(* Logix 5000 Rung export; software revision 16.04 *)

MODULES
   PBS : vendor None type None code None
   Local : vendor None type None code None
END_MODULES

TYPE ILX69PBS_UTIL_AOI :
STRUCT
   InputArray : ILX69PBS_UTIL_AOI_INPUT_ARRAY;   // Input from Module
   OutputArray : ILX69PBS_UTIL_AOI_OUTPUT_ARRAY;   // Output to Module
   InputSize : INT;
   OutputSize : INT;
   InputDataSize : INT;
   InputCopyLength : INT;
   OutputDataSize : INT;
   OutputCopyLength : INT;
   OutputCopyLastLength : INT;
   OutputConnectionSize : INT;
   UTILOutputCopyLength : INT;
   PreviousBPActivityCounter : INT;
   ReadReqMasterLengthDINT : DINT;
   AlarmReqMasterLengthDINT : DINT;
END_STRUCT
END_TYPE

TYPE ILX69PBS_UTIL_MSG_SETEXTDIAG_REQUEST :   // Slave Diagnostic Request
STRUCT
   Status : DINT;   // Slave Status
   Command : DINT;   // Message Command. Set to 0x040E
   ExtendedDiagnosticOverflow : SINT;   // Set bit 0 to indicate that more diagnostic data is available as diagnostic data can be transferred with Data below
   Reserved1 : SINT;   // Reserved
   Reserved2 : SINT;
   Reserved3 : SINT;
   ExtendedDiagData : SINT[237];   // Diagnostic Data to be transferred
END_STRUCT
END_TYPE

TYPE ILX69PBS_DPV1_READ_RESPONE_TO_MASTER :   // DPV1 Read Response to Master
STRUCT
   Initiate : BOOL;   // Initiate a response to the Masters DPV1 read request with the associated read data.
   InhibitAutoInitiate : BOOL;   // Inhibitit Automatically Initiating a response. Master Address, Slot, Index, Length and data are copied to response.
   Slot : SINT;   // Place Requested Slot Number
   Index : SINT;   // Place Requested Index
   Length : SINT;   // Place Requested Data Length
   Data : SINT[240];   // Place Requested Data
END_STRUCT
END_TYPE

TYPE ILX69PBS_DPV1_WRITE :   // DPV1 Write
STRUCT
   RequestFromMaster : ILX69PBS_DPV1_WRITE_REQ_FROM_MASTER;   // DPV1 Write Request from Master
   ResponseToMaster : ILX69PBS_DPV1_WRITE_RESPONSE_TO_MASTER;   // DPV1 Write Response to Master
   MSGStatus : ILX69PBS_MESSAGE_STATUS;   // DPV1 Write MSG Status
END_STRUCT
END_TYPE

TYPE ILX69PBS_UTIL_AOI_DEV_STATUS_REGISTER :   // Device Status Register
STRUCT
   Reserved0 : BOOL;   // Reserved
   Reserved1 : BOOL;   // Reserved
   Reserved2 : BOOL;   // Reserved
   Reserved3 : BOOL;   // Reserved
   Reserved4 : BOOL;   // Reserved
   Communication : BOOL;   // Communication
   Running : BOOL;   // Running
   Ready : BOOL;   // Ready
   Reserved5 : SINT;   // Reserved
   Reserved6 : SINT;   // Reserved
   Reserved7 : SINT;   // Reserved
END_STRUCT
END_TYPE

TYPE ILX69PBS_UTIL_MSG_DPV1_ALARM :   // DPV1 Alarm MSG Status, Source and Destination
STRUCT
   Source : ILX69PBS_UTIL_MSG_DPV1_ALARM_REQUEST;   // Source. Request from Master
   Destination : ILX69PBS_UTIL_MSG_DPV1_ALARM_RESPONSE;   // Destination. Response to Master
END_STRUCT
END_TYPE

TYPE ILX69PBS_UTIL_MSG_DPV1_WRITE_RESPONSE :   // DPV1 Write Response
STRUCT
   Status : DINT;   // Status
   Command : DINT;   // Message Command. Set to 0x0487
   SlotNumber : SINT;   // Slot Number
   Index : SINT;   // Index
   Length : SINT;   // Length
   Reserved1 : SINT;   // Reserved
   ErrorDecode : SINT;   // Error Code Classifying Fault
   ErrorCode1 : SINT;   // Detailed Error Code
   ErrorCode2 : SINT;   // User Specific Error Code
   Reserved2 : SINT;   // Reserved
   Data : SINT[240];   // Write Data
END_STRUCT
END_TYPE

TYPE ILX69PBS_UTIL_MSG_SETEXTDIAG_RESPONSE :   // Slave Diagnostic Response
STRUCT
   Status : DINT;   // Slave Status
   Command : DINT;   // Message Command. Reposnds with 0x040F
END_STRUCT
END_TYPE

TYPE ILX69PBS_CONTROL :
STRUCT
   ColdBoot : BOOL;   // Cold Boot Reset
   GetExtendedStatus : ILX69PBS_CONTROL_GETEXTENDEDDIAG;   // Get Extended Status Information Select
   SetExtendedDiagnostic : ILX69PBS_CONTROL_SETEXTENDEDDIAG;   // Set Slave Diagnostic Extended Data
END_STRUCT
END_TYPE

TYPE ILX69PBS_UTIL_MSG_DPV1_READ_REQUEST :   // DPV1 Read Request MSG Structure
STRUCT
   Status : DINT;   // Status
   Command : DINT;   // Message Command. Set to 0x0485
   SlotNumber : SINT;   // Slot Number
   Index : SINT;   // Index
   Length : SINT;   // Length
   Reserved1 : SINT;   // Reserved
   ErrorDecode : SINT;   // Error Code Classifying Fault
   ErrorCode1 : SINT;   // Detailed Error Code
   ErrorCode2 : SINT;   // User Specific Error Code
   Reserved2 : SINT;   // Reserved
   Data : SINT[240];   // Read Request Data
END_STRUCT
END_TYPE

TYPE ILX69PBS_DPV1_READ_REQ_FROM_MASTER :   // DPV1 Read Request from Master
STRUCT
   Indication : BOOL;   // DPV1 Read Request Indication from Master
   MasterAddress : SINT;   // Master Address requesting DPV1 Read
   Slot : SINT;   // Requested Slot Number to Read
   Index : SINT;   // Requested Index to Read
   Length : SINT;   // Requested Data Length to Read
END_STRUCT
END_TYPE

TYPE ILX69PBS_UTIL_MSG_DPV1_WRITE :   // DPV1 Write MSG Status, Source and Destination
STRUCT
   Source : ILX69PBS_UTIL_MSG_DPV1_WRITE_REQUEST;   // Source. Request from Master
   Destination : ILX69PBS_UTIL_MSG_DPV1_WRITE_RESPONSE;   // Destination. Response to Master
END_STRUCT
END_TYPE

TYPE ILX69PBS_STATUS_EXT_CONFIG :   // Extended Configuration Information
STRUCT
   Length : SINT;   // Number of valid configuration bytes
   Data : SINT[49];   // Configuration Bytes
END_STRUCT
END_TYPE

TYPE ILX69PBS_STATUS_EXT_PARAM :   // Extended Parameter Data
STRUCT
   Length : SINT;   // Number of valid parameter bytes
   Data : SINT[32];   // Parameter Bytes
END_STRUCT
END_TYPE

TYPE ILX69PBS_DPV1_ALARM_REQ_TO_MASTER :   // DPV1 Alarm Request to Master
STRUCT
   Initiate : BOOL;   // Initiate a DPV1 Alarm Request to the Master.
   SlotNumber : SINT;   // Slot Number for Alarm
   AlarmType : SINT;   // Alarm Type
   SequenceNumber : SINT;   // Sequence Number
   AdditionalAck : SINT;   // Additional Acknowledgement
   Specifier : SINT;   // Alarm Specifier
   Length : SINT;   // Alarm Data Length
   Data : SINT[58];   // Alarm Data
END_STRUCT
END_TYPE

TYPE ILX69PBS_UTIL_AOI_FW_REVISION :   // Firmware Major/Minor Revision
STRUCT
   FwMinor : SINT;   // Firmware Minor Revison
   FwMajor : SINT;   // Firmware Major Revison
   Reserved : INT;   // Reserved
END_STRUCT
END_TYPE

TYPE ILX69PBS_CONTROL_SETEXTENDEDDIAG :   // Slave Diagnostic Data
STRUCT
   Initiate : BOOL;   // Initiate Diagnostic Request
   ExtendedDiagnosticOverflow : SINT;   // Set bit 0 to indicate that more diagnostic data is available as diagnostic data can be transferred with Data below
   ExtendedDiagData : SINT[237];   // Diagnostic Data to be transferred
   MSGStatus : ILX69PBS_MESSAGE_STATUS;
END_STRUCT
END_TYPE

TYPE ILX69PBS_UTIL_MSG_DPV1_READ_RESPONSE :   // DPV1 Read Response MSG
STRUCT
   Status : DINT;   // Status
   Command : DINT;   // Should be 0x0485
   SlotNumber : SINT;   // Slot Number
   Index : SINT;   // Index
   Length : SINT;   // Length
   Reserved : SINT;   // Reserved
END_STRUCT
END_TYPE

TYPE ILX69PBS_STATUS_EXT :   // Extended Status Info
STRUCT
   NoneSelected : BOOL;   // Not Extended Data Selected
   FirmwareSelected : BOOL;   // Extended Firmware Data current in STATUS.ExtendedStatus.Firmware
   SlaveConfigSelected : BOOL;   // Extended Slave Configuration Data current in STATUS.ExtendedStatus.SlaveConfiguration
   MasterConfigSelected : BOOL;   // Extended Master Configuration Data current in STATUS.ExtendedStatus.MasterConfiguration
   ParameterDataSelected : BOOL;   // Extended Parameter Data current in STATUS.ExtendedStatus.ParameterData
   DPV1Selected : BOOL;   // Extended DPV1 Data current in STATUS.ExtendedStatus.PDV1
   Length : INT;   // Length of Extended Data
   Firmware : ILX69PBS_STATUS_EXT_FIRMWARE;   // Extended Firmware Info
   SlaveConfiguration : ILX69PBS_STATUS_EXT_CONFIG;   // Extended Slave Configuration Data
   MasterConfiguration : ILX69PBS_STATUS_EXT_CONFIG;   // Extended Master Configuration Data
   ParameterData : ILX69PBS_STATUS_EXT_PARAM;   // Extended Parameter Data
   DPV1 : ILX69PBS_STATUS_EXT_DPV1;   // Extended DPV1 Data
END_STRUCT
END_TYPE

TYPE ILX69PBS_CONTROL_GETEXTENDEDDIAG :   // Get Extended Status Select
STRUCT
   Firmware : BOOL;   // Places Extended Firmware Data into STATUS.ExtendedStatus.Firmware
   SlaveConfig : BOOL;   // Places Extended Slave Configuration Data into STATUS.ExtendedStatus.SlaveConfiguration
   MasterConfig : BOOL;   // Places Extended Master Configuration Data into STATUS.ExtendedStatus.MasterConfiguration
   ParameterData : BOOL;   // Places Extended Parameter Data into STATUS.ExtendedStatus.ParameterData
   DPV1 : BOOL;   // Places Extended DPV1 Data into STATUS.ExtendedStatus.DPV1
END_STRUCT
END_TYPE

TYPE ILX69PBS_UTIL :
STRUCT
   MSG : ILX69PBS_UTIL_MSG;   // Messages
END_STRUCT
END_TYPE

TYPE ILX69PBS_UTIL_MSG_DPV1_WRITE_REQUEST :   // DPV1 Write Request
STRUCT
   Status : DINT;   // Status 0=OK
   Command : DINT;   // Should return 0x0487
   SlotNumber : SINT;   // Slot Number
   Index : SINT;   // Index
   Length : SINT;   // Length
   Reserved1 : SINT;   // Reserved
   ErrorDecode : SINT;   // Error Code Classifying Fault
   ErrorCode1 : SINT;   // Error Code 1
   ErrorCode2 : SINT;   // Error Code 2
   Reserved2 : SINT;   // Reserved
END_STRUCT
END_TYPE

TYPE ILX69PBS_STATUS_EXT_DPV1 :   // DPV1 Extended Information
STRUCT
   StatusRequests : DINT;   // Number of Status Requests from User
   StatusMessagesSent : DINT;   // Number of Status Messages Sent
   NegativeStatusConfirmations : DINT;   // Number of Negative Status Confirmation to User
   DiagnosticRequests : DINT;   // Number of Diagnostic Requests from User
   DiagnosticMessagesSent : DINT;   // Number of Diagnostic Messages Sent
   NegativeDiagnosticConfirmations : DINT;   // Number of Negative Diagnostic Confirmations to User
   AlarmRequests : DINT;   // Number of Alarm Requests from User
   AlarmMessagesSent : DINT;   // Number of Alarm Messages Sent
   PositiveAlarmConfirmations : DINT;   // Number of Positive Alarm Confirmations to User
   NegativeAlarmConfirmations : DINT;   // Number of Negative Alarm Confirmations to User
   Requests : DINT;   // Number of Requests
   ImmediateNegativeConfirmations : DINT;   // Number of Immediate Negative Confirmations
   ReadWriteIndications : DINT;   // Number of Read/Write Indications to User
   PositiveReadWriteResponses : DINT;   // Number of Positive Read/Write Responses from User
   NegativeReadWriteResponses : DINT;   // Number of Negative Read/Write Responses from User
   AlarmAckIndications : DINT;   // Number of Alarm Acknowledge Indications
   AlarmAckResponses : DINT;   // Number of Alarm Acknowledge Responses
   AlarmAckErrors : DINT;   // Number of Alarm Acknowledge Errors
   ErrorResponses : DINT;   // Number of Error Responses from User
   UnexpectedErrorResponses : DINT;   // Number of Unexpected Responses from User
END_STRUCT
END_TYPE

TYPE ILX69PBS_UTIL_AOI_SLAVE_STATUS :   // Slave Status Information
STRUCT
   ExtStaSelect : INT;   // 0=No Extended status inform 1=Firmware version 2=Slave Config 3=Master Config 4=Parameter data 6=Reserved
   ExtStaLen : INT;   // 0=0 Byte 1=32 Byte 2=49 Byte 3=49 Byte 4=33 Byte 6=80 Byte
   Baudrate : INT;   // 12000=12MBaud 6000=6MBaud 3000=3MBaud 1500=1.5MBaud 500=500kBaud 187=187.5kBaud 93=93.75kBaud 9=9.6kBaud 0=not detected
   Busaddress : SINT;   // 0 ... 125
   UserFlags : SINT;   // D0=Parameter data changed D1=Configuration data changed D2...D7 Dont'care
   Indent : INT;   // Should be 0x0EE1
   Reserved : INT;   // Reserved
   InputDataLen : INT;   // Legnth of input data 0 ... 244
   OutputDataLen : INT;   // Length of output data 0 ... 244
   Reserved1 : INT;   // Should be 0
   Reserved2 : SINT;   // Should be 0
   Pad : SINT;   // Reserved. Should be 0
   WatchdogTime : INT;   // Current Watch dog time. 5 ... 65535ms
   IrqCounter : INT;   // Indication of bus activity. 0 ... 0xFFFF
   DPV1RWInd : SINT;   // A Read/Write Indication has been received. Bit 0 set indicates a Read. Bit 1 set indicates a Write.
   DPV1RWIndCnt : SINT;   // Increment on every new DPV1 request
   DPV1MasterAdr : SINT;   // Address of Requesting Master
   DPV1Slot : SINT;   // Requested Slot Number
   DPV1Index : SINT;   // Requested Index
   DPV1DataLen : SINT;   // Requested Data Length
   Reserved3 : SINT;   // Reserved
   Reserved4 : SINT;   // Reserved
   ExtStatusInfo : SINT[96];   // Dependent on ExtStaSelect value
END_STRUCT
END_TYPE

TYPE ILX69PBS_UTIL_MSG_DPV1_ALARM_RESPONSE :   // DPV1 Alarm Response Confirm
STRUCT
   Status : DINT;   // Status 0=OK
   Command : DINT;   // Should be 0x0485
   SlotNumber : SINT;   // Slot Number of module causing the alarm
   AlarmType : SINT;   // Type of alarm received
   SequenceNumber : SINT;   // Sequence Number
   Reserved : SINT;   // Reserved Padding byte. Set to 0.
END_STRUCT
END_TYPE

TYPE ILX69PBS_STATUS_FW_REVISION :   // Firmware Major/Minor Revision
STRUCT
   FwMinor : SINT;   // Firmware Minor Revison
   FwMajor : SINT;   // Firmware Major Revison
END_STRUCT
END_TYPE

TYPE ILX69PBS_DPV1_ALARM_RESPONSE_FROM_ILX :   // Alarm Response from ILX Module
STRUCT
   SlotNumber : SINT;   // Slot Number of module causing the alarm
   AlarmType : SINT;   // Type of alarm received
   SequenceNumber : SINT;   // Sequence Number
END_STRUCT
END_TYPE

TYPE ILX69PBS_UTIL_MSG_DPV1_ALARM_REQUEST :   // DPV1 Alarm Response Request
STRUCT
   Status : DINT;   // Status
   Command : DINT;   // Message Command. Set to 0x0480
   SlotNumber : SINT;   // Slot Number of data to be read
   AlarmType : SINT;   // Alarm Type
   SequenceNumber : SINT;   // Sequence Number
   AdditionalAck : SINT;   // Additional Acknowledgement
   Specifier : SINT;   // Alarm Specifier
   Length : SINT;   // Alarm Length
   Reserved1 : SINT;
   Reserved2 : SINT;
   Data : SINT[58];   // Alarm Data
END_STRUCT
END_TYPE

TYPE ILX69PBS_DPV1_WRITE_RESPONSE_TO_MASTER :   // DPV1 Write Response to Master
STRUCT
   Initiate : BOOL;   // Initiate a response to the Masters DPV1 write request to let the master know the write occurred.
   InhibitAutoInitiate : BOOL;   // Inhibitit Automatically Initiating a response. Master Address, Slot, Index and Length are copied to response.
   MasterAddress : SINT;   // Place Master Address
   Slot : SINT;   // Place Requested Slot Number
   Index : SINT;   // Place Requested Index
   Length : SINT;   // Place Requested Data Length
END_STRUCT
END_TYPE

TYPE ILX69PBS_DPV1 :   // DPV1
STRUCT
   Read : ILX69PBS_DPV1_READ;
   Write : ILX69PBS_DPV1_WRITE;
   Alarm : ILX69PBS_DPV1_ALARM;
   RWCount : SINT;
END_STRUCT
END_TYPE

TYPE ILX69PBS_DPV1_READ :   // DPV1 Read
STRUCT
   RequestFromMaster : ILX69PBS_DPV1_READ_REQ_FROM_MASTER;   // DPV1 Read Request from Master
   ResponseToMaster : ILX69PBS_DPV1_READ_RESPONE_TO_MASTER;   // DPV1 Read Response to Master
   MSGStatus : ILX69PBS_MESSAGE_STATUS;   // DPV1 Read MSG Status
END_STRUCT
END_TYPE

TYPE ILX69PBS_UTIL_AOI_OUTPUT_ARRAY :
STRUCT
   DeviceCommandRegister : ILX69PBS_UTIL_AOI_DEV_COMMAND_REGISTER;   // Command Register
   OutputData : SINT[244];   // PROFIBUS Input data.
END_STRUCT
END_TYPE

TYPE ILX69PBS_DPV1_WRITE_REQ_FROM_MASTER :   // DPV1 Write Request from Master
STRUCT
   Indication : BOOL;   // DPV1 Write Request Indication from Master
   MasterAddress : SINT;   // Master Address requesting DPV1 Write
   Slot : SINT;   // Request Slot Number to Write to
   Index : SINT;   // Requested Index to Write to
   Length : SINT;   // Requested Data Length to Write to
   Data : SINT[240];   // Requested Data to Write
END_STRUCT
END_TYPE

TYPE ILX69PBS_UTIL_MSG :   // MSG Instructions
STRUCT
   DPV1Read : ILX69PBS_UTIL_MSG_DPV1_READ;
   DPV1Write : ILX69PBS_UTIL_MSG_DPV1_WRITE;
   DPV1Alarm : ILX69PBS_UTIL_MSG_DPV1_ALARM;
   SetExtDiag : ILX69PBS_UTIL_MSG_SETEXTDIAG;
END_STRUCT
END_TYPE

TYPE ILX69PBS_DATA :
STRUCT
   Output : SINT[244];   // Input Data. Profibus Output Data
   Input : SINT[244];   // Output Data. Profibus Input Data.
END_STRUCT
END_TYPE

TYPE ILX69PBS_MESSAGE_STATUS :   // Message Status
STRUCT
   Done : BOOL;   // Message transmitted. Response is available
   Error : BOOL;   // Last message transmitted with an error
   DoneCount : DINT;   // Response OK Count
   ErrorCount : DINT;   // Error Count
END_STRUCT
END_TYPE

TYPE ILX69PBS_DPV1_ALARM :   // DPV1 Alarm Request
STRUCT
   RequestToMaster : ILX69PBS_DPV1_ALARM_REQ_TO_MASTER;   // DPV1 Alarm Request to Master
   ResponseFromILX : ILX69PBS_DPV1_ALARM_RESPONSE_FROM_ILX;   // DPV1 Alarm Response from ILX Module
   MSGStatus : ILX69PBS_MESSAGE_STATUS;   // DPV1 Alarm MSG Status
END_STRUCT
END_TYPE

TYPE ILX69PBS_STATUS_EXT_FIRMWARE :   // Extended Firmware Information
STRUCT
   Version : ILX69PBS_STATUS_EXT_FIRMWARE_VERSION;   // Firmware Version
   Name : ILX69PBS_STATUS_EXT_FIRMWARE_NAME;   // Firmware Name
   Date : ILX69PBS_STATUS_EXT_FIRMWARE_DATE;   // Firmware Date
END_STRUCT
END_TYPE

TYPE ILX69PBS_UTIL_AOI_DEV_COMMAND_REGISTER :   // Device Command Register
STRUCT
   Reserved0 : BOOL;   // Reserved
   Reserved1 : BOOL;   // Reserved
   Reserved2 : BOOL;   // Reserved
   Reserved3 : BOOL;   // Reserved
   Reserved4 : BOOL;   // Reserved
   Reserved5 : BOOL;   // Application Not Ready
   Reserved6 : BOOL;   // Init ( Warm boot )
   Reset : BOOL;   // Reset ( Cold boot )
   Reserved7 : SINT;   // Reserved
   Reserved8 : SINT;   // Reserved
   ExtStaSelect : SINT;   // Extended Status Information Select 1=Firmware 2=Slave Config 3=Master Config 4=Parameter Data 5+ Reserved
END_STRUCT
END_TYPE

TYPE ILX69PBS_STATUS_EXT_FIRMWARE_VERSION :   // Version
STRUCT
   Major : INT;   // Major
   Minor : INT;   // Minor
   Build : INT;   // Build
   Revision : INT;   // Revision
END_STRUCT
END_TYPE

TYPE ILX69PBS_MODULEDEF :   // ILX69-PBS PROFIBUS Slave Module Definition
STRUCT
   PROFIBUSDATA : ILX69PBS_DATA;   // Profibus Data
   DPV1 : ILX69PBS_DPV1;   // DPV1
   STATUS : ILX69PBS_STATUS;   // Module Status
   CONTROL : ILX69PBS_CONTROL;   // Module Control
   UTIL : ILX69PBS_UTIL;   // Util. Not used by user.
END_STRUCT
END_TYPE

TYPE ILX69PBS_UTIL_AOI_INPUT_ARRAY :   // Input Array
STRUCT
   DeviceStatusRegister : ILX69PBS_UTIL_AOI_DEV_STATUS_REGISTER;   // Device Status
   FirmwareRev : ILX69PBS_UTIL_AOI_FW_REVISION;   // Firmware Revision and Block Size
   SlaveStatus : ILX69PBS_UTIL_AOI_SLAVE_STATUS;   // Slave Status
   InputData : SINT[244];   // PROFIBUS Output data.
END_STRUCT
END_TYPE

TYPE ILX69PBS_STATUS :   // Status
STRUCT
   Communication : BOOL;   // Profibus communication is started and the module is engaged in cyclic data exchange with the master
   Running : BOOL;   // Running. Module is ready for communication.
   Ready : BOOL;   // Ready. Module is operational.
   Address : SINT;   // Slave Bus Address
   Identification : INT;   // Slave Identification Number. Should be 0x0EE1
   BaudRate : INT;   // Baud Rate 12000=12M 6000=6M 3000=3M 1500=1.5M 500=500k 187=187.5k 93=93.75k 9=9.6k 0=not detected
   FirmwareRevision : ILX69PBS_STATUS_FW_REVISION;   // Firmware Revision
   ExtendedStatus : ILX69PBS_STATUS_EXT;   // Extended Status Information
   ParameterDataChange : BOOL;   // Parameter Data Changed
   ConfigurationDataChange : BOOL;   // Configuration Data Changed
   InputDataLength : INT;   // Input Data Length 0-244
   OutputDataLength : INT;   // Output Data Length 0-244
   WatchdogTime : INT;   // Current Watchdog Time
   ProfibusActivityCounter : INT;   // Profibus Activity Counter
END_STRUCT
END_TYPE

TYPE ILX69PBS_STATUS_EXT_FIRMWARE_NAME :   // Name
STRUCT
   Name : SINT[64];   // Firmware Name
END_STRUCT
END_TYPE

TYPE ILX69PBS_STATUS_EXT_FIRMWARE_DATE :   // Date
STRUCT
   Month : SINT;   // Month
   Day : SINT;   // Day
   Year : INT;   // Year
END_STRUCT
END_TYPE

TYPE ILX69PBS_UTIL_MSG_DPV1_READ :   // DPV1 Read MSG Status, Source and Destination
STRUCT
   Source : ILX69PBS_UTIL_MSG_DPV1_READ_REQUEST;   // Source. Request from Master
   Destination : ILX69PBS_UTIL_MSG_DPV1_READ_RESPONSE;   // Destination. Response to Master
END_STRUCT
END_TYPE

TYPE ILX69PBS_UTIL_MSG_SETEXTDIAG :   // Slave Diagnostic Data
STRUCT
   Source : ILX69PBS_UTIL_MSG_SETEXTDIAG_REQUEST;   // Request
   Destination : ILX69PBS_UTIL_MSG_SETEXTDIAG_RESPONSE;
END_STRUCT
END_TYPE

ADD_ON_INSTRUCTION AOIILX69PBS   (* revision 1.1, vendor ProSoft Technology Inc., ExecutePrescan *)
// Add-On instruction for ILX69-PBS ProSoft module
// Revision note:
// v1.1 - Fixed found typo errors in UDT
// v1.0 - Initial Revision
VAR_IN_OUT
   ILX69PBS : ILX69PBS_MODULEDEF; {required}
   Connection_Input : INT[190]; {required}
        [0].5   // Communication
        [0].6   // Running
        [0].7   // Ready
   Connection_Output : INT[124]; {required}
   MSGDPV1Read : MESSAGE; {required}   // DPV1 Read Message
   MSGDPV1Write : MESSAGE; {required}   // DPV1 Write Message
   MSGDPV1Alarm : MESSAGE; {required}   // DPV1 Alarm Request Message
   MSGSetExtDiag : MESSAGE; {required}   // Slave Diagnostic Request Message
END_VAR
VAR
   UTIL : ILX69PBS_UTIL_AOI;
END_VAR

ROUTINE Logic   (* ladder *)
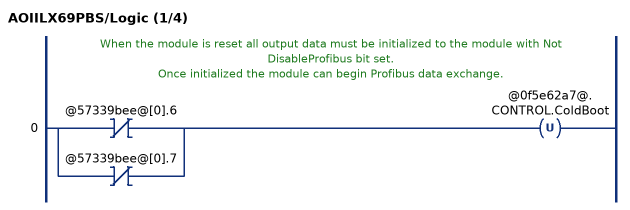
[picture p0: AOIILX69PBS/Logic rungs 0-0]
   // When the module is reset all output data must be initialized to the module with Not DisableProfibus bit set.
   // Once initialized the module can begin Profibus data exchange.
   0: [XIO(@57339bee@[0].6) ,XIO(@57339bee@[0].7) ]OTU(@0f5e62a7@.CONTROL.ColdBoot);
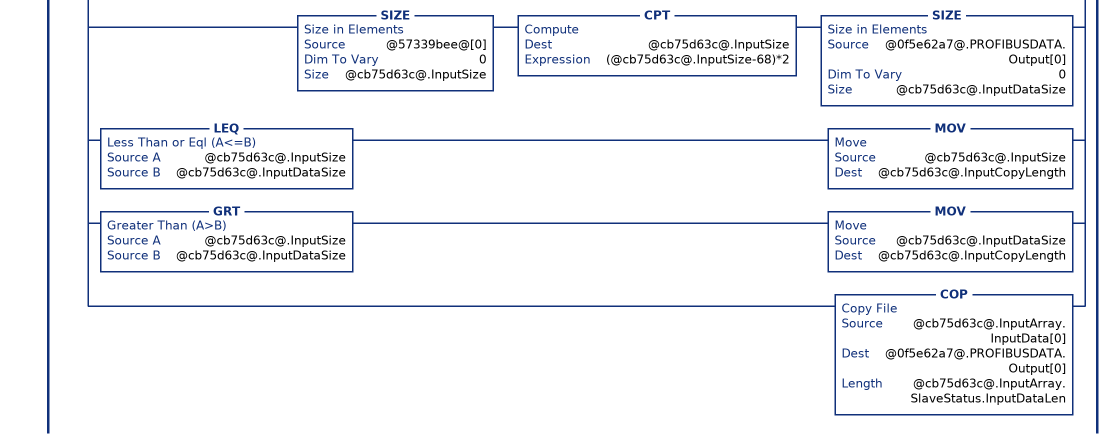
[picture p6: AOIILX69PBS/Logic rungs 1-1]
   // Handle Input Data
   1: COP(@57339bee@[0],@cb75d63c@.InputArray,1)[MOV(@cb75d63c@.InputArray.SlaveStatus.IrqCounter,@cb75d63c@.PreviousBPActivityCounter) ,[[XIC(@cb75d63c@.InputArray.DeviceStatusRegister.Communication) XIO(@0f5e62a7@.STATUS.Communication) OTL(@0f5e62a7@.STATUS.Communication) ,XIO(@cb75d63c@.InputArray.DeviceStatusRegister.Communication) XIC(@0f5e62a7@.STATUS.Communication) OTU(@0f5e62a7@.STATUS.Communication) ] ,[XIC(@cb75d63c@.InputArray.DeviceStatusRegister.Running) XIO(@0f5e62a7@.STATUS.Running) OTL(@0f5e62a7@.STATUS.Running) ,XIO(@cb75d63c@.InputArray.DeviceStatusRegister.Running) XIC(@0f5e62a7@.STATUS.Running) OTU(@0f5e62a7@.STATUS.Running) ] ,[XIC(@cb75d63c@.InputArray.DeviceStatusRegister.Ready) XIO(@0f5e62a7@.STATUS.Ready) OTL(@0f5e62a7@.STATUS.Ready) ,XIO(@cb75d63c@.InputArray.DeviceStatusRegister.Ready) XIC(@0f5e62a7@.STATUS.Ready) OTU(@0f5e62a7@.STATUS.Ready) ] ] ,COP(@cb75d63c@.InputArray.FirmwareRev,@0f5e62a7@.STATUS.FirmwareRevision,1) ,LIM(0,@cb75d63c@.InputArray.SlaveStatus.ExtStaSelect,6) [OTU(@0f5e62a7@.STATUS.ExtendedStatus.NoneSelected) ,OTU(@0f5e62a7@.STATUS.ExtendedStatus.FirmwareSelected) ,OTU(@0f5e62a7@.STATUS.ExtendedStatus.SlaveConfigSelected) ,OTU(@0f5e62a7@.STATUS.ExtendedStatus.MasterConfigSelected) ,OTU(@0f5e62a7@.STATUS.ExtendedStatus.ParameterDataSelected) ,OTU(@0f5e62a7@.STATUS.ExtendedStatus.DPV1Selected) ] [XIO(@cb75d63c@.InputArray.SlaveStatus.ExtStaSelect.2) XIO(@cb75d63c@.InputArray.SlaveStatus.ExtStaSelect.1) XIO(@cb75d63c@.InputArray.SlaveStatus.ExtStaSelect.0) OTL(@0f5e62a7@.STATUS.ExtendedStatus.NoneSelected) ,XIO(@cb75d63c@.InputArray.SlaveStatus.ExtStaSelect.2) XIO(@cb75d63c@.InputArray.SlaveStatus.ExtStaSelect.1) XIC(@cb75d63c@.InputArray.SlaveStatus.ExtStaSelect.0) OTL(@0f5e62a7@.STATUS.ExtendedStatus.FirmwareSelected) ,XIO(@cb75d63c@.InputArray.SlaveStatus.ExtStaSelect.2) XIC(@cb75d63c@.InputArray.SlaveStatus.ExtStaSelect.1) XIO(@cb75d63c@.InputArray.SlaveStatus.ExtStaSelect.0) OTL(@0f5e62a7@.STATUS.ExtendedStatus.SlaveConfigSelected) ,XIO(@cb75d63c@.InputArray.SlaveStatus.ExtStaSelect.2) XIC(@cb75d63c@.InputArray.SlaveStatus.ExtStaSelect.1) XIC(@cb75d63c@.InputArray.SlaveStatus.ExtStaSelect.0) OTL(@0f5e62a7@.STATUS.ExtendedStatus.MasterConfigSelected) ,XIC(@cb75d63c@.InputArray.SlaveStatus.ExtStaSelect.2) XIO(@cb75d63c@.InputArray.SlaveStatus.ExtStaSelect.1) XIO(@cb75d63c@.InputArray.SlaveStatus.ExtStaSelect.0) OTL(@0f5e62a7@.STATUS.ExtendedStatus.ParameterDataSelected) ,XIC(@cb75d63c@.InputArray.SlaveStatus.ExtStaSelect.2) XIC(@cb75d63c@.InputArray.SlaveStatus.ExtStaSelect.1) XIO(@cb75d63c@.InputArray.SlaveStatus.ExtStaSelect.0) OTL(@0f5e62a7@.STATUS.ExtendedStatus.DPV1Selected) ] ,[MOV(@cb75d63c@.InputArray.SlaveStatus.ExtStaLen,@0f5e62a7@.STATUS.ExtendedStatus.Length) ,XIC(@0f5e62a7@.STATUS.ExtendedStatus.FirmwareSelected) [COP(@cb75d63c@.InputArray.SlaveStatus.ExtStatusInfo[0],@0f5e62a7@.STATUS.ExtendedStatus.Firmware.Version.Major,4) ,COP(@cb75d63c@.InputArray.SlaveStatus.ExtStatusInfo[12],@0f5e62a7@.STATUS.ExtendedStatus.Firmware.Name.Name[0],64) ,COP(@cb75d63c@.InputArray.SlaveStatus.ExtStatusInfo[10],@0f5e62a7@.STATUS.ExtendedStatus.Firmware.Date.Month,1) COP(@cb75d63c@.InputArray.SlaveStatus.ExtStatusInfo[11],@0f5e62a7@.STATUS.ExtendedStatus.Firmware.Date.Day,1) COP(@cb75d63c@.InputArray.SlaveStatus.ExtStatusInfo[8],@0f5e62a7@.STATUS.ExtendedStatus.Firmware.Date.Year,1) ] ,XIC(@0f5e62a7@.STATUS.ExtendedStatus.SlaveConfigSelected) [MOV(@0f5e62a7@.STATUS.ExtendedStatus.Length,@0f5e62a7@.STATUS.ExtendedStatus.SlaveConfiguration.Length) ,COP(@cb75d63c@.InputArray.SlaveStatus.ExtStatusInfo[0],@0f5e62a7@.STATUS.ExtendedStatus.SlaveConfiguration.Data[0],@0f5e62a7@.STATUS.ExtendedStatus.Length) ] ,XIC(@0f5e62a7@.STATUS.ExtendedStatus.MasterConfigSelected) [MOV(@0f5e62a7@.STATUS.ExtendedStatus.Length,@0f5e62a7@.STATUS.ExtendedStatus.MasterConfiguration.Length) ,COP(@cb75d63c@.InputArray.SlaveStatus.ExtStatusInfo[0],@0f5e62a7@.STATUS.ExtendedStatus.MasterConfiguration.Data[0],@0f5e62a7@.STATUS.ExtendedStatus.Length) ] ,XIC(@0f5e62a7@.STATUS.ExtendedStatus.ParameterDataSelected) [MOV(@0f5e62a7@.STATUS.ExtendedStatus.Length,@0f5e62a7@.STATUS.ExtendedStatus.ParameterData.Length) ,COP(@cb75d63c@.InputArray.SlaveStatus.ExtStatusInfo[0],@0f5e62a7@.STATUS.ExtendedStatus.ParameterData.Data[0],@0f5e62a7@.STATUS.ExtendedStatus.Length) ] ,XIC(@0f5e62a7@.STATUS.ExtendedStatus.DPV1Selected) CPT(@0f5e62a7@.STATUS.ExtendedStatus.Length,@cb75d63c@.InputArray.SlaveStatus.ExtStaLen/4) COP(@cb75d63c@.InputArray.SlaveStatus.ExtStatusInfo[0],@0f5e62a7@.STATUS.ExtendedStatus.DPV1.StatusRequests,@0f5e62a7@.STATUS.ExtendedStatus.Length) MOV(@cb75d63c@.InputArray.SlaveStatus.ExtStaLen,@0f5e62a7@.STATUS.ExtendedStatus.Length) ] ,MOV(@cb75d63c@.InputArray.SlaveStatus.Baudrate,@0f5e62a7@.STATUS.BaudRate) MOV(@cb75d63c@.InputArray.SlaveStatus.Busaddress,@0f5e62a7@.STATUS.Address) ,[[XIC(@cb75d63c@.InputArray.SlaveStatus.UserFlags.0) XIO(@0f5e62a7@.STATUS.ParameterDataChange) OTL(@0f5e62a7@.STATUS.ParameterDataChange) ,XIO(@cb75d63c@.InputArray.SlaveStatus.UserFlags.0) XIC(@0f5e62a7@.STATUS.ParameterDataChange) OTU(@0f5e62a7@.STATUS.ParameterDataChange) ] ,[XIC(@cb75d63c@.InputArray.SlaveStatus.UserFlags.1) XIO(@0f5e62a7@.STATUS.ConfigurationDataChange) OTL(@0f5e62a7@.STATUS.ConfigurationDataChange) ,XIO(@cb75d63c@.InputArray.SlaveStatus.UserFlags.1) XIC(@0f5e62a7@.STATUS.ConfigurationDataChange) OTU(@0f5e62a7@.STATUS.ConfigurationDataChange) ] ] ,MOV(@cb75d63c@.InputArray.SlaveStatus.Indent,@0f5e62a7@.STATUS.Identification) ,MOV(@cb75d63c@.InputArray.SlaveStatus.InputDataLen,@0f5e62a7@.STATUS.InputDataLength) MOV(@cb75d63c@.InputArray.SlaveStatus.OutputDataLen,@0f5e62a7@.STATUS.OutputDataLength) ,MOV(@cb75d63c@.InputArray.SlaveStatus.WatchdogTime,@0f5e62a7@.STATUS.WatchdogTime) MOV(@cb75d63c@.InputArray.SlaveStatus.IrqCounter,@0f5e62a7@.STATUS.ProfibusActivityCounter) ,[[XIC(@cb75d63c@.InputArray.SlaveStatus.DPV1RWInd.0) XIO(@0f5e62a7@.DPV1.Read.RequestFromMaster.Indication) OTL(@0f5e62a7@.DPV1.Read.RequestFromMaster.Indication) ,XIO(@cb75d63c@.InputArray.SlaveStatus.DPV1RWInd.0) XIC(@0f5e62a7@.DPV1.Read.RequestFromMaster.Indication) OTU(@0f5e62a7@.DPV1.Read.RequestFromMaster.Indication) ] ,[XIC(@cb75d63c@.InputArray.SlaveStatus.DPV1RWInd.1) XIO(@0f5e62a7@.DPV1.Write.RequestFromMaster.Indication) OTL(@0f5e62a7@.DPV1.Write.RequestFromMaster.Indication) ,XIO(@cb75d63c@.InputArray.SlaveStatus.DPV1RWInd.1) XIC(@0f5e62a7@.DPV1.Write.RequestFromMaster.Indication) OTU(@0f5e62a7@.DPV1.Write.RequestFromMaster.Indication) ] ] ,MOV(@cb75d63c@.InputArray.SlaveStatus.DPV1RWIndCnt,@0f5e62a7@.DPV1.RWCount) ,[XIC(@0f5e62a7@.DPV1.Read.RequestFromMaster.Indication) COP(@cb75d63c@.InputArray.SlaveStatus.DPV1MasterAdr,@0f5e62a7@.DPV1.Read.RequestFromMaster.MasterAddress,4) ,XIC(@0f5e62a7@.DPV1.Write.RequestFromMaster.Indication) [COP(@cb75d63c@.InputArray.SlaveStatus.DPV1MasterAdr,@0f5e62a7@.DPV1.Write.RequestFromMaster.MasterAddress,4) ,COP(@cb75d63c@.InputArray.SlaveStatus.ExtStatusInfo[0],@0f5e62a7@.DPV1.Write.RequestFromMaster.Data[0],@0f5e62a7@.DPV1.Write.RequestFromMaster.Length) ] ] ,[SIZE(@57339bee@[0],0,@cb75d63c@.InputSize) CPT(@cb75d63c@.InputSize,(@cb75d63c@.InputSize-68)*2) SIZE(@0f5e62a7@.PROFIBUSDATA.Output[0],0,@cb75d63c@.InputDataSize) ,[LEQ(@cb75d63c@.InputSize,@cb75d63c@.InputDataSize) MOV(@cb75d63c@.InputSize,@cb75d63c@.InputCopyLength) ,GRT(@cb75d63c@.InputSize,@cb75d63c@.InputDataSize) MOV(@cb75d63c@.InputDataSize,@cb75d63c@.InputCopyLength) ] ] ,COP(@cb75d63c@.InputArray.InputData[0],@0f5e62a7@.PROFIBUSDATA.Output[0],@cb75d63c@.InputArray.SlaveStatus.InputDataLen) ];
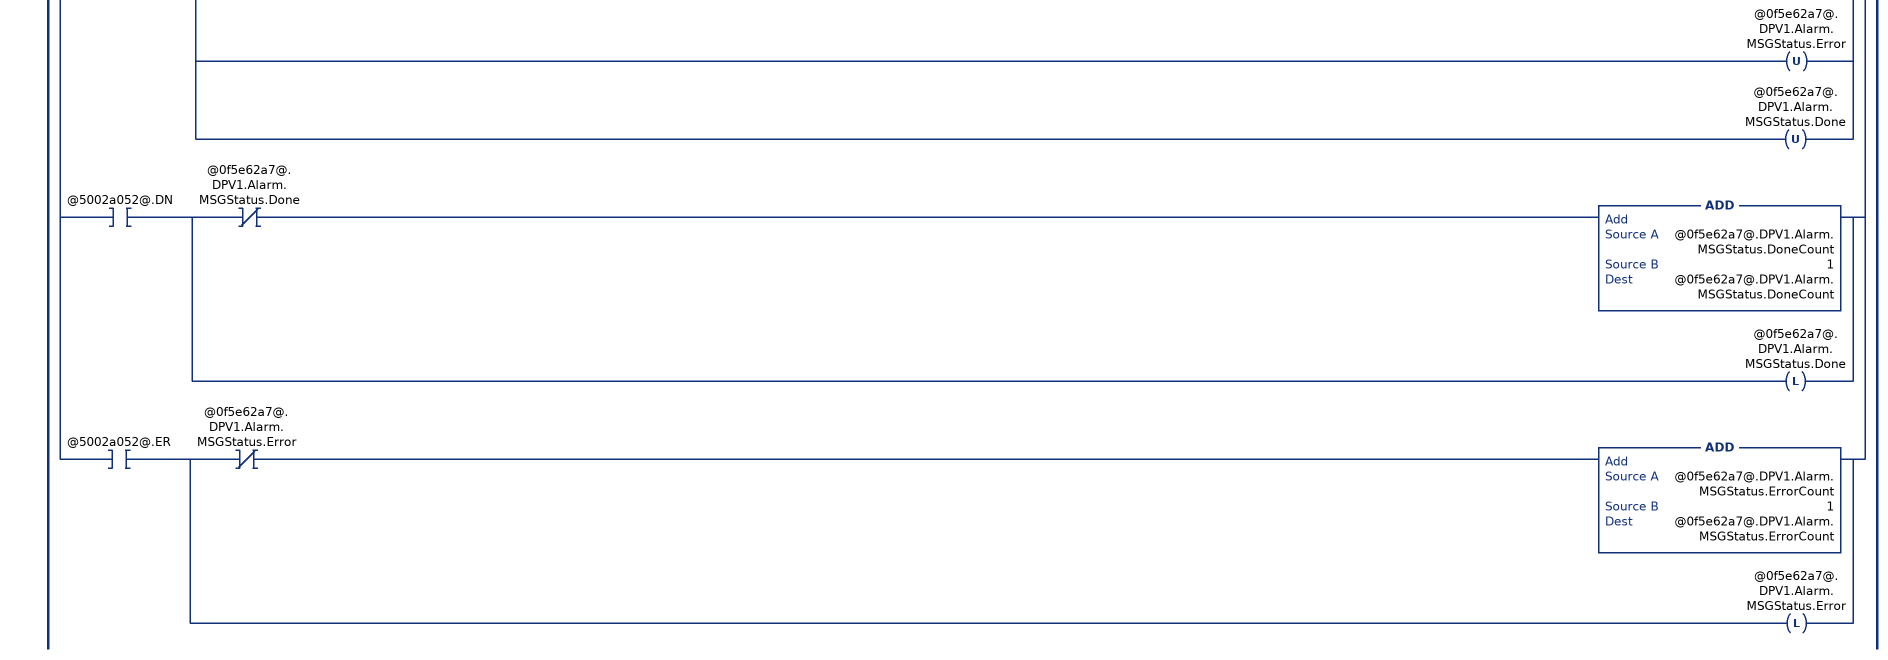
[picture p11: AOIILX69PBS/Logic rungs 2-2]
   // Message Handling
   2: [[XIC(@0f5e62a7@.CONTROL.SetExtendedDiagnostic.Initiate) [XIC(@c76ac9cd@.DN) ,XIC(@c76ac9cd@.ER) ] [MOV(16#040E,@0f5e62a7@.UTIL.MSG.SetExtDiag.Source.Command) ,MOV(@0f5e62a7@.CONTROL.SetExtendedDiagnostic.ExtendedDiagnosticOverflow,@0f5e62a7@.UTIL.MSG.SetExtDiag.Source.ExtendedDiagnosticOverflow) ,COP(@0f5e62a7@.CONTROL.SetExtendedDiagnostic.ExtendedDiagData[0],@0f5e62a7@.UTIL.MSG.SetExtDiag.Source.ExtendedDiagData[0],237) ,MSG(@c76ac9cd@) ,OTU(@0f5e62a7@.CONTROL.SetExtendedDiagnostic.Initiate) ,OTU(@0f5e62a7@.CONTROL.SetExtendedDiagnostic.MSGStatus.Error) ,OTU(@0f5e62a7@.CONTROL.SetExtendedDiagnostic.MSGStatus.Done) ] ,XIC(@c76ac9cd@.DN) [XIO(@0f5e62a7@.CONTROL.SetExtendedDiagnostic.MSGStatus.Done) ADD(@0f5e62a7@.CONTROL.SetExtendedDiagnostic.MSGStatus.DoneCount,1,@0f5e62a7@.CONTROL.SetExtendedDiagnostic.MSGStatus.DoneCount) ,OTL(@0f5e62a7@.CONTROL.SetExtendedDiagnostic.MSGStatus.Done) ] ,XIC(@c76ac9cd@.ER) [XIO(@0f5e62a7@.CONTROL.SetExtendedDiagnostic.MSGStatus.Error) ADD(@0f5e62a7@.CONTROL.SetExtendedDiagnostic.MSGStatus.ErrorCount,1,@0f5e62a7@.CONTROL.SetExtendedDiagnostic.MSGStatus.ErrorCount) ,OTL(@0f5e62a7@.CONTROL.SetExtendedDiagnostic.MSGStatus.Error) ] ] ,[XIC(@0f5e62a7@.DPV1.Read.RequestFromMaster.Indication) [XIC(@ec32f5b8@.DN) ,XIC(@ec32f5b8@.ER) ] [XIC(@0f5e62a7@.DPV1.Read.ResponseToMaster.Initiate) ,XIO(@0f5e62a7@.DPV1.Read.ResponseToMaster.InhibitAutoInitiate) [COP(@0f5e62a7@.DPV1.Read.RequestFromMaster.Slot,@0f5e62a7@.UTIL.MSG.DPV1Read.Source.SlotNumber,3) ,COP(@0f5e62a7@.DPV1.Read.ResponseToMaster.Data[0],@0f5e62a7@.UTIL.MSG.DPV1Read.Source.Data[0],@0f5e62a7@.DPV1.Read.RequestFromMaster.Length) ] ] [MVM(@0f5e62a7@.DPV1.Read.RequestFromMaster.Length,16#FF,@cb75d63c@.ReadReqMasterLengthDINT) CPT(@ec32f5b8@.REQ_LEN,16+@cb75d63c@.ReadReqMasterLengthDINT) [LES(@ec32f5b8@.REQ_LEN,16) MOV(16,@ec32f5b8@.REQ_LEN) ,GRT(@ec32f5b8@.REQ_LEN,256) MOV(256,@ec32f5b8@.REQ_LEN) ] ,[MOV(16#0485,@0f5e62a7@.UTIL.MSG.DPV1Read.Source.Command) ,MSG(@ec32f5b8@) ,OTU(@0f5e62a7@.DPV1.Read.ResponseToMaster.Initiate) ,OTU(@0f5e62a7@.DPV1.Read.MSGStatus.Error) ,OTU(@0f5e62a7@.DPV1.Read.MSGStatus.Done) ] ] ,XIC(@ec32f5b8@.DN) [XIO(@0f5e62a7@.DPV1.Read.MSGStatus.Done) ADD(@0f5e62a7@.DPV1.Read.MSGStatus.DoneCount,1,@0f5e62a7@.DPV1.Read.MSGStatus.DoneCount) ,OTL(@0f5e62a7@.DPV1.Read.MSGStatus.Done) ] ,XIC(@ec32f5b8@.ER) [XIO(@0f5e62a7@.DPV1.Read.MSGStatus.Error) ADD(@0f5e62a7@.DPV1.Read.MSGStatus.ErrorCount,1,@0f5e62a7@.DPV1.Read.MSGStatus.ErrorCount) ,OTL(@0f5e62a7@.DPV1.Read.MSGStatus.Error) ] ] ,[XIC(@0f5e62a7@.DPV1.Write.RequestFromMaster.Indication) [XIC(@ad53215b@.DN) ,XIC(@ad53215b@.ER) ] [XIC(@0f5e62a7@.DPV1.Write.ResponseToMaster.Initiate) ,XIO(@0f5e62a7@.DPV1.Write.ResponseToMaster.InhibitAutoInitiate) [COP(@0f5e62a7@.DPV1.Write.RequestFromMaster.Slot,@0f5e62a7@.UTIL.MSG.DPV1Write.Source.SlotNumber,3) ,COP(@0f5e62a7@.UTIL.MSG.DPV1Write.Destination.Data[0],@0f5e62a7@.DPV1.Write.RequestFromMaster.Data[0],@0f5e62a7@.DPV1.Write.RequestFromMaster.Length) ] ] [MOV(16#0487,@0f5e62a7@.UTIL.MSG.DPV1Write.Source.Command) ,MSG(@ad53215b@) ,OTU(@0f5e62a7@.DPV1.Write.ResponseToMaster.Initiate) ,OTU(@0f5e62a7@.DPV1.Write.MSGStatus.Error) ,OTU(@0f5e62a7@.DPV1.Write.MSGStatus.Done) ] ,XIC(@ad53215b@.DN) [XIO(@0f5e62a7@.DPV1.Write.MSGStatus.Done) ADD(@0f5e62a7@.DPV1.Write.MSGStatus.DoneCount,1,@0f5e62a7@.DPV1.Write.MSGStatus.DoneCount) ,OTL(@0f5e62a7@.DPV1.Write.MSGStatus.Done) ] ,XIC(@ad53215b@.ER) [XIO(@0f5e62a7@.DPV1.Write.MSGStatus.Error) ADD(@0f5e62a7@.DPV1.Write.MSGStatus.ErrorCount,1,@0f5e62a7@.DPV1.Write.MSGStatus.ErrorCount) ,OTL(@0f5e62a7@.DPV1.Write.MSGStatus.Error) ] ] ,[XIC(@0f5e62a7@.DPV1.Alarm.RequestToMaster.Initiate) [MVM(@0f5e62a7@.DPV1.Alarm.RequestToMaster.Length,16#FF,@cb75d63c@.AlarmReqMasterLengthDINT) CPT(@5002a052@.REQ_LEN,16+@cb75d63c@.AlarmReqMasterLengthDINT) [LES(@5002a052@.REQ_LEN,16) MOV(16,@5002a052@.REQ_LEN) ,GRT(@5002a052@.REQ_LEN,74) MOV(74,@5002a052@.REQ_LEN) ] ,MOV(16#0480,@0f5e62a7@.UTIL.MSG.DPV1Alarm.Source.Command) COP(@0f5e62a7@.DPV1.Alarm.RequestToMaster.SlotNumber,@0f5e62a7@.UTIL.MSG.DPV1Alarm.Source.SlotNumber,6) COP(@0f5e62a7@.DPV1.Alarm.RequestToMaster.Data[0],@0f5e62a7@.UTIL.MSG.DPV1Alarm.Source.Data[0],@0f5e62a7@.DPV1.Alarm.RequestToMaster.Length) ,MSG(@5002a052@) ,OTU(@0f5e62a7@.DPV1.Alarm.RequestToMaster.Initiate) ,OTU(@0f5e62a7@.DPV1.Alarm.MSGStatus.Error) ,OTU(@0f5e62a7@.DPV1.Alarm.MSGStatus.Done) ] ,XIC(@5002a052@.DN) [XIO(@0f5e62a7@.DPV1.Alarm.MSGStatus.Done) ADD(@0f5e62a7@.DPV1.Alarm.MSGStatus.DoneCount,1,@0f5e62a7@.DPV1.Alarm.MSGStatus.DoneCount) ,OTL(@0f5e62a7@.DPV1.Alarm.MSGStatus.Done) ] ,XIC(@5002a052@.ER) [XIO(@0f5e62a7@.DPV1.Alarm.MSGStatus.Error) ADD(@0f5e62a7@.DPV1.Alarm.MSGStatus.ErrorCount,1,@0f5e62a7@.DPV1.Alarm.MSGStatus.ErrorCount) ,OTL(@0f5e62a7@.DPV1.Alarm.MSGStatus.Error) ] ] ];
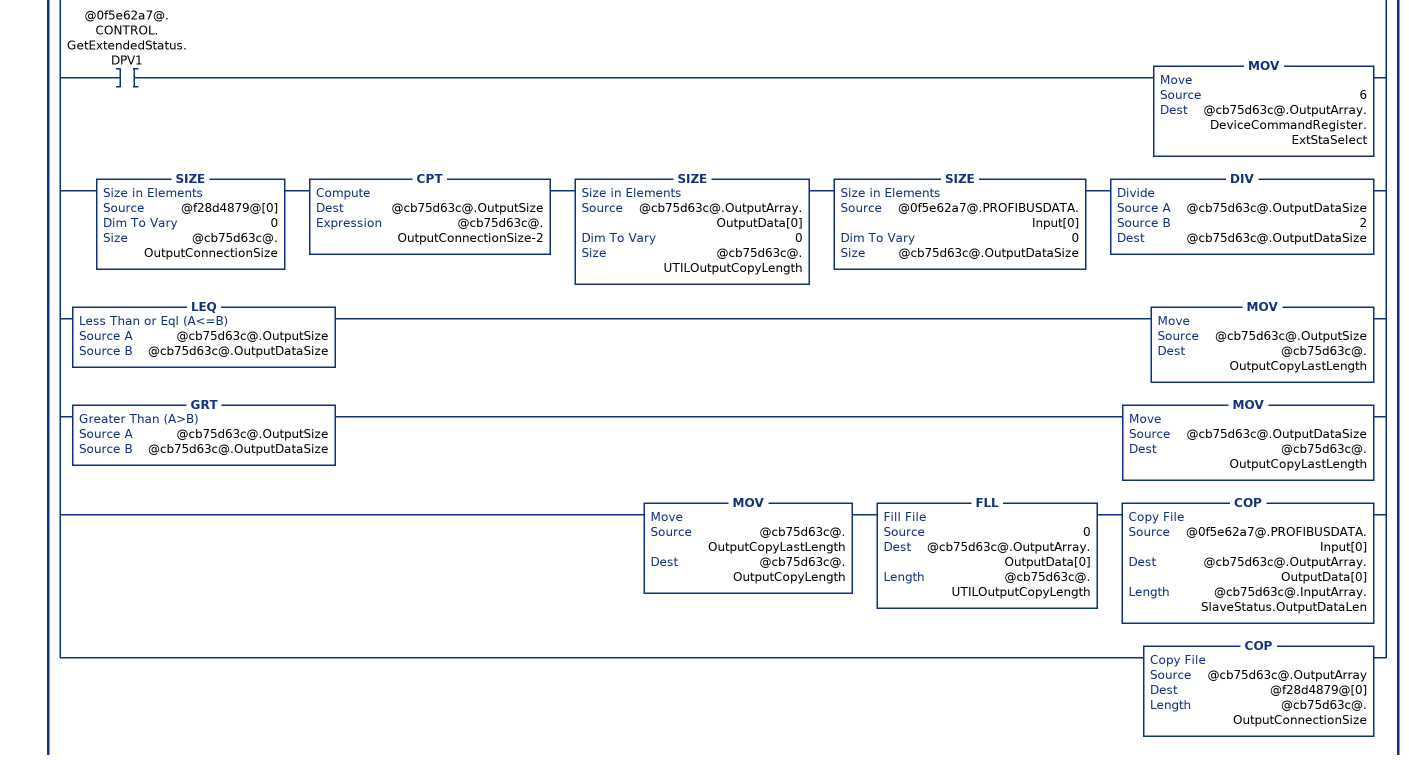
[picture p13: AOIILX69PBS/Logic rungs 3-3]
   // Handle Output Data
   3: [[[XIC(@0f5e62a7@.CONTROL.ColdBoot) XIO(@cb75d63c@.OutputArray.DeviceCommandRegister.Reset) OTL(@cb75d63c@.OutputArray.DeviceCommandRegister.Reset) ,XIO(@0f5e62a7@.CONTROL.ColdBoot) XIC(@cb75d63c@.OutputArray.DeviceCommandRegister.Reset) OTU(@cb75d63c@.OutputArray.DeviceCommandRegister.Reset) ] ,[XIO(@0f5e62a7@.CONTROL.GetExtendedStatus.Firmware) XIO(@0f5e62a7@.CONTROL.GetExtendedStatus.SlaveConfig) XIO(@0f5e62a7@.CONTROL.GetExtendedStatus.MasterConfig) XIO(@0f5e62a7@.CONTROL.GetExtendedStatus.ParameterData) MOV(0,@cb75d63c@.OutputArray.DeviceCommandRegister.ExtStaSelect) ,XIC(@0f5e62a7@.CONTROL.GetExtendedStatus.Firmware) MOV(1,@cb75d63c@.OutputArray.DeviceCommandRegister.ExtStaSelect) ,XIC(@0f5e62a7@.CONTROL.GetExtendedStatus.SlaveConfig) MOV(2,@cb75d63c@.OutputArray.DeviceCommandRegister.ExtStaSelect) ,XIC(@0f5e62a7@.CONTROL.GetExtendedStatus.MasterConfig) MOV(3,@cb75d63c@.OutputArray.DeviceCommandRegister.ExtStaSelect) ,XIC(@0f5e62a7@.CONTROL.GetExtendedStatus.ParameterData) MOV(4,@cb75d63c@.OutputArray.DeviceCommandRegister.ExtStaSelect) ,XIC(@0f5e62a7@.CONTROL.GetExtendedStatus.DPV1) MOV(6,@cb75d63c@.OutputArray.DeviceCommandRegister.ExtStaSelect) ] ] ,[SIZE(@f28d4879@[0],0,@cb75d63c@.OutputConnectionSize) CPT(@cb75d63c@.OutputSize,@cb75d63c@.OutputConnectionSize-2) SIZE(@cb75d63c@.OutputArray.OutputData[0],0,@cb75d63c@.UTILOutputCopyLength) SIZE(@0f5e62a7@.PROFIBUSDATA.Input[0],0,@cb75d63c@.OutputDataSize) DIV(@cb75d63c@.OutputDataSize,2,@cb75d63c@.OutputDataSize) ,[LEQ(@cb75d63c@.OutputSize,@cb75d63c@.OutputDataSize) MOV(@cb75d63c@.OutputSize,@cb75d63c@.OutputCopyLastLength) ,GRT(@cb75d63c@.OutputSize,@cb75d63c@.OutputDataSize) MOV(@cb75d63c@.OutputDataSize,@cb75d63c@.OutputCopyLastLength) ] ] ,MOV(@cb75d63c@.OutputCopyLastLength,@cb75d63c@.OutputCopyLength) FLL(0,@cb75d63c@.OutputArray.OutputData[0],@cb75d63c@.UTILOutputCopyLength) COP(@0f5e62a7@.PROFIBUSDATA.Input[0],@cb75d63c@.OutputArray.OutputData[0],@cb75d63c@.InputArray.SlaveStatus.OutputDataLen) ,COP(@cb75d63c@.OutputArray,@f28d4879@[0],@cb75d63c@.OutputConnectionSize) ];
END_ROUTINE

ROUTINE Prescan   (* ladder *)
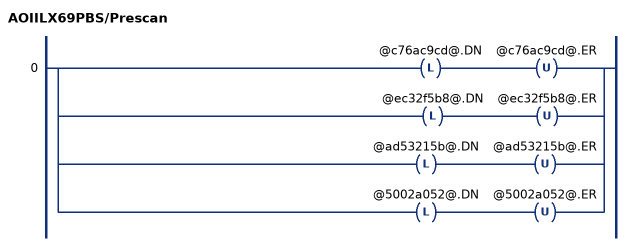
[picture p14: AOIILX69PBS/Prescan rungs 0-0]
   0: [OTL(@c76ac9cd@.DN) OTU(@c76ac9cd@.ER) ,OTL(@ec32f5b8@.DN) OTU(@ec32f5b8@.ER) ,OTL(@ad53215b@.DN) OTU(@ad53215b@.ER) ,OTL(@5002a052@.DN) OTU(@5002a052@.ER) ];
END_ROUTINE
END_ADD_ON_INSTRUCTION

VAR_GLOBAL   (* controller tags *)
   ILX69PBS : ILX69PBS_MODULEDEF;
   Local:1:I : PS:ILX69_PBS:I:0;
   Local:1:O : PS:ILX69_PBS:O:0;
   ILX69PBS_MSGDPV1Alarm : MESSAGE;   // DPV1 Alarm Request Message
        MessageParameters(MessageType := CIP Generic, RequestedLength := 74, ConnectedFlag := 2, ConnectionPath := PBS, ServiceCode := 16#0064, ObjectType := 16#0065, TargetObject := 2, LocalElement := ILX69PBS.UTIL.MSG.DPV1Alarm.Source, DestinationTag := ILX69PBS.UTIL.MSG.DPV1Alarm.Destination)
   ILX69PBS_MSGDPV1Write : MESSAGE;   // DPV1 Write Message
        MessageParameters(MessageType := CIP Generic, RequestedLength := 32, ConnectedFlag := 2, ConnectionPath := PBS, ServiceCode := 16#0064, ObjectType := 16#0065, TargetObject := 2, LocalElement := ILX69PBS.UTIL.MSG.DPV1Write.Source, DestinationTag := ILX69PBS.UTIL.MSG.DPV1Write.Destination)
   ILX69PBS_MSGSetExtDiag : MESSAGE;   // Slave Diagnostic Request Message
        MessageParameters(MessageType := CIP Generic, RequestedLength := 38, ConnectedFlag := 2, ConnectionPath := PBS, ServiceCode := 16#0064, ObjectType := 16#0065, TargetObject := 2, LocalElement := ILX69PBS.UTIL.MSG.SetExtDiag.Source, DestinationTag := ILX69PBS.UTIL.MSG.SetExtDiag.Destination)
   AOIILX69PBS : AOIILX69PBS;
   ILX69PBS_MSGDPV1Read : MESSAGE;   // DPV1 Read Message
        MessageParameters(MessageType := CIP Generic, RequestedLength := 26, ConnectedFlag := 2, ConnectionPath := PBS, ServiceCode := 16#0064, ObjectType := 16#0065, TargetObject := 2, LocalElement := ILX69PBS.UTIL.MSG.DPV1Read.Source, DestinationTag := ILX69PBS.UTIL.MSG.DPV1Read.Destination)
END_VAR

PROGRAM MainProgram

ROUTINE MainRoutine   (* ladder *)
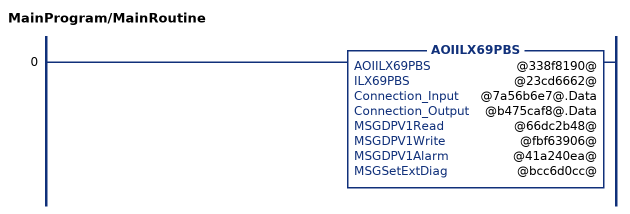
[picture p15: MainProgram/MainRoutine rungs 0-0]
   0: AOIILX69PBS(@338f8190@,@23cd6662@,@7a56b6e7@.Data,@b475caf8@.Data,@66dc2b48@,@fbf63906@,@41a240ea@,@bcc6d0cc@);
END_ROUTINE
END_PROGRAM
